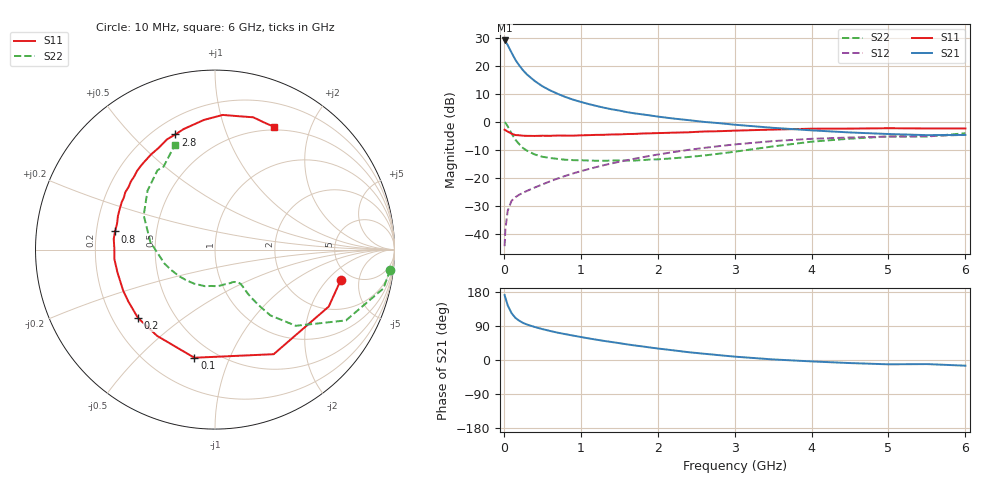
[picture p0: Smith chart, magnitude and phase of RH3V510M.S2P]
! SIEMENS Small Signal Semiconductors
! BFR106
! Si NPN RF Bipolar Junction Transistor in SOT23
! VCE = 3.5 V  IC = 10 mA
! Common Emitter S-Parameters:  August  1996
# GHz  S  MA  R  50
!  f  S11  S21  S12  S22
! GHz  MAG  ANG  MAG  ANG  MAG  ANG  MAG  ANG
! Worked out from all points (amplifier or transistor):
!   36 points, 10 MHz to 6 GHz, reference 50 ohm
!   highest |S21| = 29.0 dB at 10 MHz (marker M1)
!   |S21| within 3 dB of that: start of sweep to 75.33 MHz
!   unconditionally stable (mu >= 1): 484.1 MHz to 2.103 GHz; 5.12 GHz to end of sweep
!   at 250 MHz: K = 0.72, MSG = 21.9 dB, |S12| = -25.4 dB
!   at 1.4 GHz: K = 1.09, MAG = 7.8 dB, |S12| = -14.9 dB
!   at 6 GHz: K = 1.01, MAG = -0.7 dB, |S12| = -4.7 dB
!   S11 on the Smith chart (normalised r, x): 10 MHz: 4.06, -2.87; 100 MHz: 0.39, -0.75; 200 MHz: 0.31, -0.35; 800 MHz: 0.28, +0.08; 2.8 GHz: 0.28, +0.67; 6 GHz: 0.46, +1.49
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0.01  0.7211 -13.6  28.32 171.3  0.006 84.8  0.9828 -6.6
0.02  0.7087 -26.6  27.46 164.3  0.0119 77.7  0.9626 -13.0
0.05  0.6682 -60.7  23.46 144.4  0.0257 63.2  0.8296 -28.4
0.1  0.6134 -100.8  17.2 123.7  0.0388 51.5  0.619 -43.3
0.15  0.5788 -123.9  12.79 111.1  0.045 46.4  0.4793 -49.9
0.2  0.5737 -138.5  10.15 103.7  0.0498 45.7  0.3975 -51.8
0.25  0.5628 -149.0  8.285 97.8  0.0539 46.8  0.3385 -52.9
0.3  0.5604 -155.9  7.003 93.7  0.0582 48.6  0.3055 -53.3
0.4  0.5582 -166.9  5.361 87.2  0.0668 51.8  0.2612 -53.1
0.5  0.563 -174.6  4.32 81.6  0.0759 54.6  0.2375 -53.2
0.6  0.5611 179.1  3.642 76.7  0.0862 57.1  0.2254 -54.7
0.7  0.5674 173.9  3.154 72.1  0.0969 58.8  0.2171 -56.9
0.8  0.5659 169.7  2.771 68.2  0.108 59.7  0.2096 -59.2
1.1  0.5768 157.2  2.076 57.1  0.1426 61.3  0.2033 -69.0
1.3  0.5847 150.3  1.786 50.5  0.1676 61.0  0.2009 -76.7
1.6  0.6031 141.0  1.485 41.3  0.2053 59.4  0.2036 -90.5
2.2  0.6385 124.0  1.143 25.6  0.2869 53.5  0.2225 -121.4
2.8  0.6784 109.0  0.944 12.7  0.3672 44.7  0.2694 -155.1
3.5  0.725 94.9  0.779 1.5  0.4518 33.3  0.363 173.3
4.5  0.7548 79.9  0.644 -8.1  0.5238 16.2  0.4991 138.9
5.5  0.7586 68.0  0.577 -10.8  0.5551 5.1  0.5437 121.8
6  0.7591 64.5  0.582 -15.0  0.584 -2.6  0.6238 111.1
